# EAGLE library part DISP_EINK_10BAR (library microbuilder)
eInk 10-Bar Display
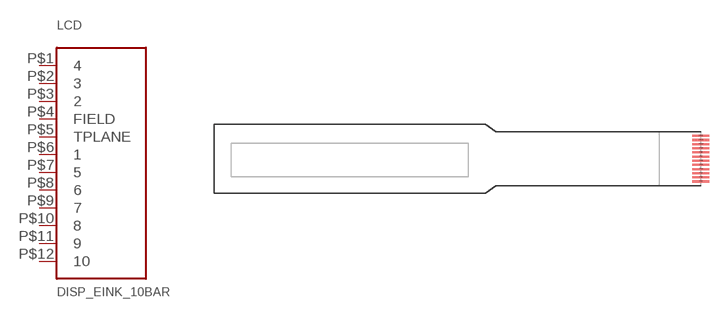
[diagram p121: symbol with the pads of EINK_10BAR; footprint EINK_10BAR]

Designator prefix LCD

## DISP_EINK_10BAR  [EINK_10BAR]
P$1  4
P$2  3
P$3  2
P$4  FIELD
P$5  TPLANE
P$6  1
P$7  5
P$8  6
P$9  7
P$10  8
P$11  9
P$12  10

## Footprint EINK_10BAR (pad centres in mm)
smd 2 x 0.25: P$1 0,1.4; P$2 0,1.9; P$3 0,2.4; P$4 0,2.9; P$5 0,3.4; P$6 0,3.9; P$7 0,4.4; P$8 0,4.9; P$9 0,5.4; P$10 0,5.9; P$11 0,6.4; P$12 0,6.9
